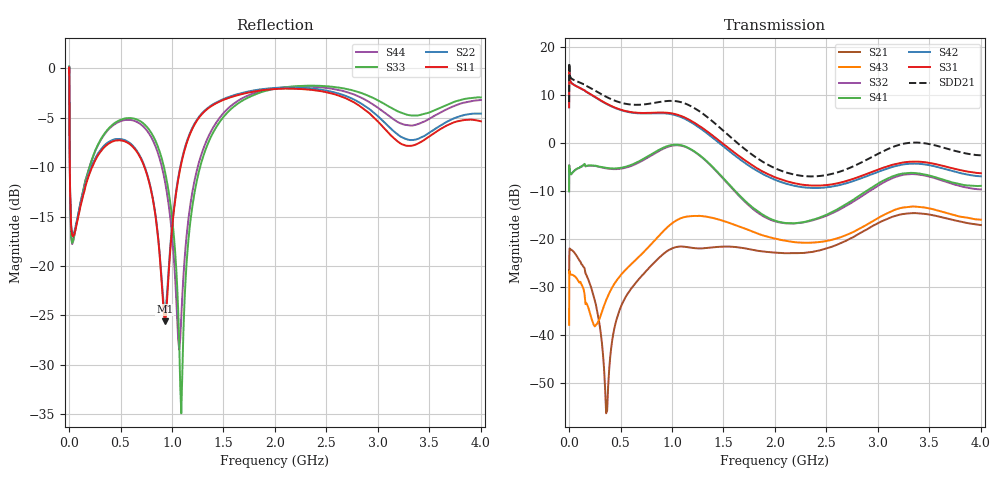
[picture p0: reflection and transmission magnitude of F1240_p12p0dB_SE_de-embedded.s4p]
! Integrated Device Technology
! Corporate Headquarters
! 6024 Silver Creek Valley Road
! San Jose, CA 95138  USA
! Phone:  1-408-284-8200
! Toll Free:  1-800-223-1366
! Webpage:  http://www.idt.com/
! Timing and RF Division
! 515 Groton Road, Suite 102
! Westford, MA 01886-6024
! Device:  F1240
! Description: Dual Intermediate Frequency Digital Variable Gain Amplifier
! Frequency:  10.0 -  500.00 MHz
! Package:  5x5 mm QFN Plastic Package: 32 pin
! Ports:  8 RF, 20 DC
!  Pin  1  = GA3 / Data  Pin 17  = RF OUT_B+
!  Pin  2  = GA4 / CLK  Pin 18  = RF OUT_B-
!  Pin  3  = GA5  Pin 19  = STBY_B
!  Pin  4  = VMODE  Pin 20  = Ground
!  Pin  5  = No Connect  Pin 21  = Ground
!  Pin  6  = GB5  Pin 22  = STB_A
!  Pin  7  = GB4  Pin 23  = RF OUT_A-  = Port 4
!  Pin  8  = GB3  Pin 24  = RF OUT_A+  = Port 3
!  Pin  9  = GB2  Pin 25  = GA0
!  Pin 10  = GB1  Pin 26  = ISET_A
!  Pin 11  = RF IN_B+  Pin 27  = VCC
!  Pin 12  = RF IN_B-  Pin 28  = Ground
!  Pin 13  = Ground  Pin 29  = RF IN_A-  = Port 2
!  Pin 14  = VCC  Pin 30  = RF IN_A+  = Port 1
!  Pin 15  = ISET_B  Pin 31  = GA1
!  Pin 16  = GB0  Pin 32  = GA2 / CSb
! Gain  = +19.5 dB
! State  = 1
! Voltage  = +5.00 V
! Current  = 85.292 mA (one channel only)
! Temperture  =  +25 C
! Test Date  =  2017-10-18
! Board  =  EB4031
! Data:  The device was measured on a custom evaluation board which has
!  individual transmission lines to the RF pins.  Data was collected
!  using a calibrated network analyzer.  The evaluation board was
!  de-embedded using Automatic Fixture Removal.
!  The reference plane is the edge of the package pin.
!  Only Channel A was measured.
!  This data is in single-ended operation.  If your needs are balanced
!  or differential S-parameters then this file needs to be used a
!  linear simulator.
! File Date:  2017-11-10  MJV
! Note:
!  Integrated Device Technology supplies this data as a sample of measured
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# Hz S dB R 100
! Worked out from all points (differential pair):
!   410 points, 500 kHz to 4 GHz, reference 100 ohm
!   strongest paths, dB at 500 kHz, 930 MHz, 1.96 GHz, 2.98 GHz, 4 GHz:
!     S31: 7.4, 6.3, -6.8, -5.7, -6.3
!     S42: 7.4, 6.1, -7.3, -6.2, -7.0
!     S41: -10.1, -0.9, -15.9, -8.8, -9.0
!     S32: -10.1, -1.1, -16.1, -9.2, -9.7
!     S43: -37.9, -18.1, -19.7, -16.0, -16.0
!     S21: -26.6, -22.9, -22.8, -17.0, -17.1
!   taken as a pair (ports 1,2 in; 3,4 out), SDD21 dB: 8.5, 8.7, -4.9, -2.5, -2.6
!   lowest |S11| = -25.6 dB at 930 MHz (marker M1), VSWR 1.11, Z = 109 + j6.48 ohm
!   |S11| at or under -10 dB: 7.457 MHz to 223.5 MHz (216.1 MHz wide, 187 % of centre); 733 MHz to 1.082 GHz (349.2 MHz wide, 38.5 % of centre)
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500000  -0.38 -5.8  -26.58 -1.9  -27.26 79.5  -59.46 68.5
        -26.60 -2.0  -0.38 -5.8  -59.37 67.4  -27.27 80.6
        7.41 -105.2  -10.07 69.8  -0.47 1.3  -37.98 -127.8
        -10.11 70.9  7.39 -104.0  -37.92 -127.6  -0.48 3.6
3000000  -3.65 -57.5  -22.94 10.0  -17.32 19.5  -44.18 63.7
         -22.92 10.0  -3.62 -57.5  -44.16 63.5  -17.32 19.7
         15.28 -175.7  -5.46 -6.8  -3.19 -53.1  -26.73 55.6
         -5.41 -6.7  15.27 -175.5  -26.71 55.6  -3.25 -52.8
2e8  -10.62 -124.7  -29.12 -90.4  -19.76 -51.2  -34.19 12.6
     -29.25 -88.8  -10.39 -126.0  -34.16 12.9  -19.78 -51.3
     10.25 109.4  -4.75 -41.7  -9.93 -87.8  -34.01 -124.4
     -4.70 -42.0  10.21 108.7  -35.28 -123.1  -9.93 -87.0
5.4e8  -7.37 -178.2  -33.35 -1.6  -21.24 -109.2  -28.25 -58.6
       -32.51 -6.8  -7.25 -179.5  -28.38 -56.9  -21.38 -109.5
       6.67 24.7  -5.24 -109.2  -5.07 -155.1  -28.01 25.3
       -5.04 -110.7  6.59 23.7  -26.64 18.1  -5.22 -155.0
9.3e8  -25.58 34.3  -22.57 -75.1  -18.91 169.0  -24.32 -150.9
       -22.93 -84.4  -24.65 31.9  -24.62 -145.3  -19.27 168.4
       6.30 -71.4  -1.09 159.2  -10.36 140.6  -19.16 -58.5
       -0.88 154.9  6.14 -73.2  -18.10 -67.3  -11.35 142.7
1.52e9  -3.09 -148.9  -21.12 145.2  -24.81 31.0  -26.21 73.2
        -21.61 148.5  -3.01 -148.8  -26.02 79.0  -25.86 30.6
        -0.60 126.7  -8.02 -24.2  -4.67 -135.0  -16.82 135.0
        -7.86 -29.6  -1.12 125.5  -16.41 130.9  -4.30 -138.1
4e9  -5.35 -154.1  -17.20 68.9  -21.09 -53.9  -20.28 -48.0
     -17.14 68.4  -4.57 -149.4  -22.23 -28.9  -23.88 -44.9
     -6.33 14.8  -9.70 -108.6  -2.93 -137.8  -16.01 89.3
     -8.97 -120.9  -6.98 23.7  -16.02 62.2  -3.19 -143.9
